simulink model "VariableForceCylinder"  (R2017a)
settings: Solver=VariableStepAuto  StartTime=0.0  StopTime=10  RelTol=1e-3
libraries: fl_lib x8, nesl_utility x4, sh_lib x3

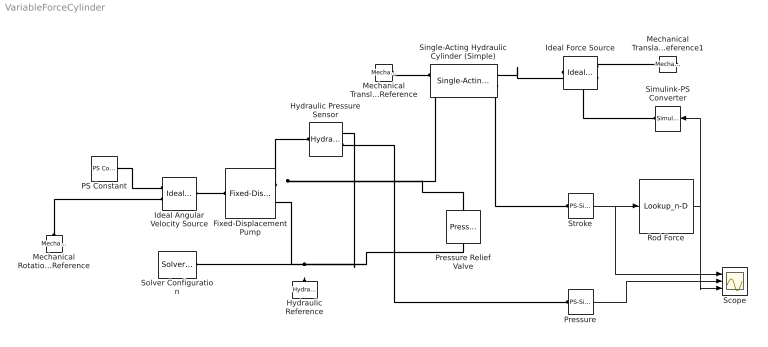
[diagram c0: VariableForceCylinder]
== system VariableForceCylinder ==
  Fixed-Displacement Pump : sh_lib/Pumps and Motors/Fixed-Displacement Pump  D=10 cm^3/rev  loss_spec=1  w_nominal=188 rad/s  pr_nominal=400 bar  visc_nominal=18 cSt  dens_nominal=900 kg/m^3  efficiency_vol=0.92  no_load_torque=0.05 N*m  torque_pressure_coeff=0.6e-6 N*m/Pa  p_diff_eff_TLU=[100000.0, 1000000.0, 2000000.0] Pa  omega_eff_TLU=[25.0, 50.0, 100.0, 200.0, 300.0, 400.0] rad/s  vol_eff_TLU=[0.816, 0.908, 0.954, 0.977, 0.981, 0.984; 0.325, 0.663, 0.831, 0.916, 0.925, 0.946; 0.137, 0.568, 0.78, 0.892, 0.893, 0.91]  mech_eff_TLU=[0.996, 0.996, 0.996, 0.996, 0.996, 0.996; 0.988, 0.989, 0.989, 0.989, 0.989, 0.99; 0.981, 0.981, 0.982, 0.982, 0.983, 0.984]  p_diff_loss_TLU=[100000.0, 1000000.0, 2000000.0] Pa  omega_loss_TLU=[25.0, 50.0, 100.0, 200.0, 300.0, 400.0] rad/s  vol_loss_TLU=[0.023, 0.023, 0.023, 0.023, 0.0285, 0.032; 0.0844, 0.0842, 0.0845, 0.084, 0.1125, 0.108; 0.1079, 0.108, 0.11, 0.108, 0.1605, 0.18] * 1e-3 m^3/s  mech_loss_TLU=[0.002, 0.002, 0.002, 0.002, 0.002, 0.002; 0.0607, 0.0556, 0.0556, 0.0556, 0.0556, 0.0505; 0.1937, 0.1937, 0.1833, 0.1833, 0.1729, 0.1626] N*m  pressure_threshold=1e5 Pa  omega_threshold=10 rad/s  quadrant_check=0  pressure_check=0  min_valid_pressure=0 Pa  vol_eff_min=1e-3  vol_eff_max=1  mech_eff_min=1e-3  mech_eff_max=1
  Hydraulic Pressure Sensor : fl_lib/Hydraulic/Hydraulic Sensors/Hydraulic Pressure Sensor
  Hydraulic Reference : fl_lib/Hydraulic/Hydraulic Elements/Hydraulic Reference
  Ideal Angular Velocity Source : fl_lib/Mechanical/Mechanical Sources/Ideal Angular Velocity Source
  Ideal Force Source : fl_lib/Mechanical/Mechanical Sources/Ideal Force Source
  Mechanical Rotational Reference : fl_lib/Mechanical/Rotational Elements/Mechanical Rotational Reference
  Mechanical Translational Reference : fl_lib/Mechanical/Translational Elements/Mechanical Translational Reference
  Mechanical Translational Reference1 : fl_lib/Mechanical/Translational Elements/Mechanical Translational Reference
  PS Constant : fl_lib/Physical Signals/Sources/PS Constant  constant=10
  Pressure : nesl_utility/PS-Simulink Converter  PhysicalDomain=network_engine_domain  SubClassName=ps_output  LeftPortType=input  RightPortType=output  PseudoPeriodic=off  Frequencies=[]  Unit=bar  AffineConversion=off
  Pressure Relief Valve : sh_lib/Valves/Pressure Control Valves/Pressure Relief Valve  area_max=1e-4 m^2  pres_set=70 bar  reg_range=5e5 Pa  C_d=0.7  A_leak=1e-12 m^2  lam_spec=1  B_lam=0.999  Re_cr=12  dynamic=0  tau=0.1 s  area_init=1e-12 m^2
  Rod Force : Lookup_n-D  NumberOfTableDimensions=1  BreakpointsForDimension1=[0,30,80]  Table=[2000,2500,6500]  InternalRulePriority=Speed  RndMeth=Simplest
  Scope : Scope  NumInputPorts=3
  Simulink-PS Converter : nesl_utility/Simulink-PS Converter  PhysicalDomain=network_engine_domain  SubClassName=ps_input  LeftPortType=input  RightPortType=output  PseudoPeriodic=off  Frequencies=[]  NoiseDistribution=none  NoiseParameters=[]  Unit=N  AffineConversion=off  FilteringAndDerivatives=provide  SimscapeFilterOrder=1  InputFilterTimeConstant=0.001  UdotUserProvided=0
  Single-Acting Hydraulic Cylinder (Simple) : sh_lib/Hydraulic Cylinders/Single-Acting Hydraulic Cylinder (Simple)  area=1256 mm^2  stroke=90 mm  init_pos=0 mm  penetr_coeff=1e12 s*N/m^2  or=1
  Solver Configuration : nesl_utility/Solver Configuration  PhysicalDomain=network_engine_domain  SubClassName=solver  LeftPortType=input  RightPortType=generic  Accelerate=off  Tones=[]  Harmonics=[]  SimulateNoise=off  Profile=off  UseLocalSampling=off  EnableSwitchedLinearOptims=on  FrequencyDomain=off  UseCCode=off  RelTol=0.001  AbsTol=1e-06  MinStep=1e-09  ToWorkspace=off  RevertToSquareIcSolve=off  NumHomotopyIterations=100  PhasorMode=off  PhasorModeNumHarmonics=1  OverrideAbsTol=off  DoDC=off  ResidualTolerance=1e-09  UseLocalSolver=off  LocalSolverChoice=NE_BACKWARD_EULER_ADVANCER  LocalSolverSampleTime=0.001  DoFixedCost=off  MaxNonlinIter=3  MaxModeIter=2  LinearAlgebra=Sparse  DelaysMemoryBudget=1024  AutomaticFiltering=on  FilteringTimeConstant=0.001
  Stroke : nesl_utility/PS-Simulink Converter  PhysicalDomain=network_engine_domain  SubClassName=ps_output  LeftPortType=input  RightPortType=output  PseudoPeriodic=off  Frequencies=[]  Unit=mm  AffineConversion=off
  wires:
  Stroke/1 -> Rod Force/1, Scope/1
  Pressure/1 -> Scope/2
  Rod Force/1 -> Scope/3, Simulink-PS Converter/1
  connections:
  Hydraulic Reference/LConn1 -- Hydraulic Pressure Sensor/RConn1 -- Pressure Relief Valve/RConn1 -- Fixed-Displacement Pump/RConn2 -- Solver Configuration/RConn1
  Mechanical Translational Reference/LConn1 -- Single-Acting Hydraulic Cylinder (Simple)/LConn1
  Single-Acting Hydraulic Cylinder (Simple)/RConn2 -- Stroke/LConn1
  Ideal Angular Velocity Source/LConn1 -- Fixed-Displacement Pump/LConn1
  Mechanical Rotational Reference/LConn1 -- Ideal Angular Velocity Source/RConn2
  PS Constant/RConn1 -- Ideal Angular Velocity Source/RConn1
  Hydraulic Pressure Sensor/RConn2 -- Pressure/LConn1
  Fixed-Displacement Pump/RConn1 -- Pressure Relief Valve/LConn1 -- Single-Acting Hydraulic Cylinder (Simple)/LConn2 -- Hydraulic Pressure Sensor/LConn1
  Single-Acting Hydraulic Cylinder (Simple)/RConn1 -- Ideal Force Source/RConn2
  Ideal Force Source/LConn1 -- Mechanical Translational Reference1/LConn1
  Ideal Force Source/RConn1 -- Simulink-PS Converter/RConn1
